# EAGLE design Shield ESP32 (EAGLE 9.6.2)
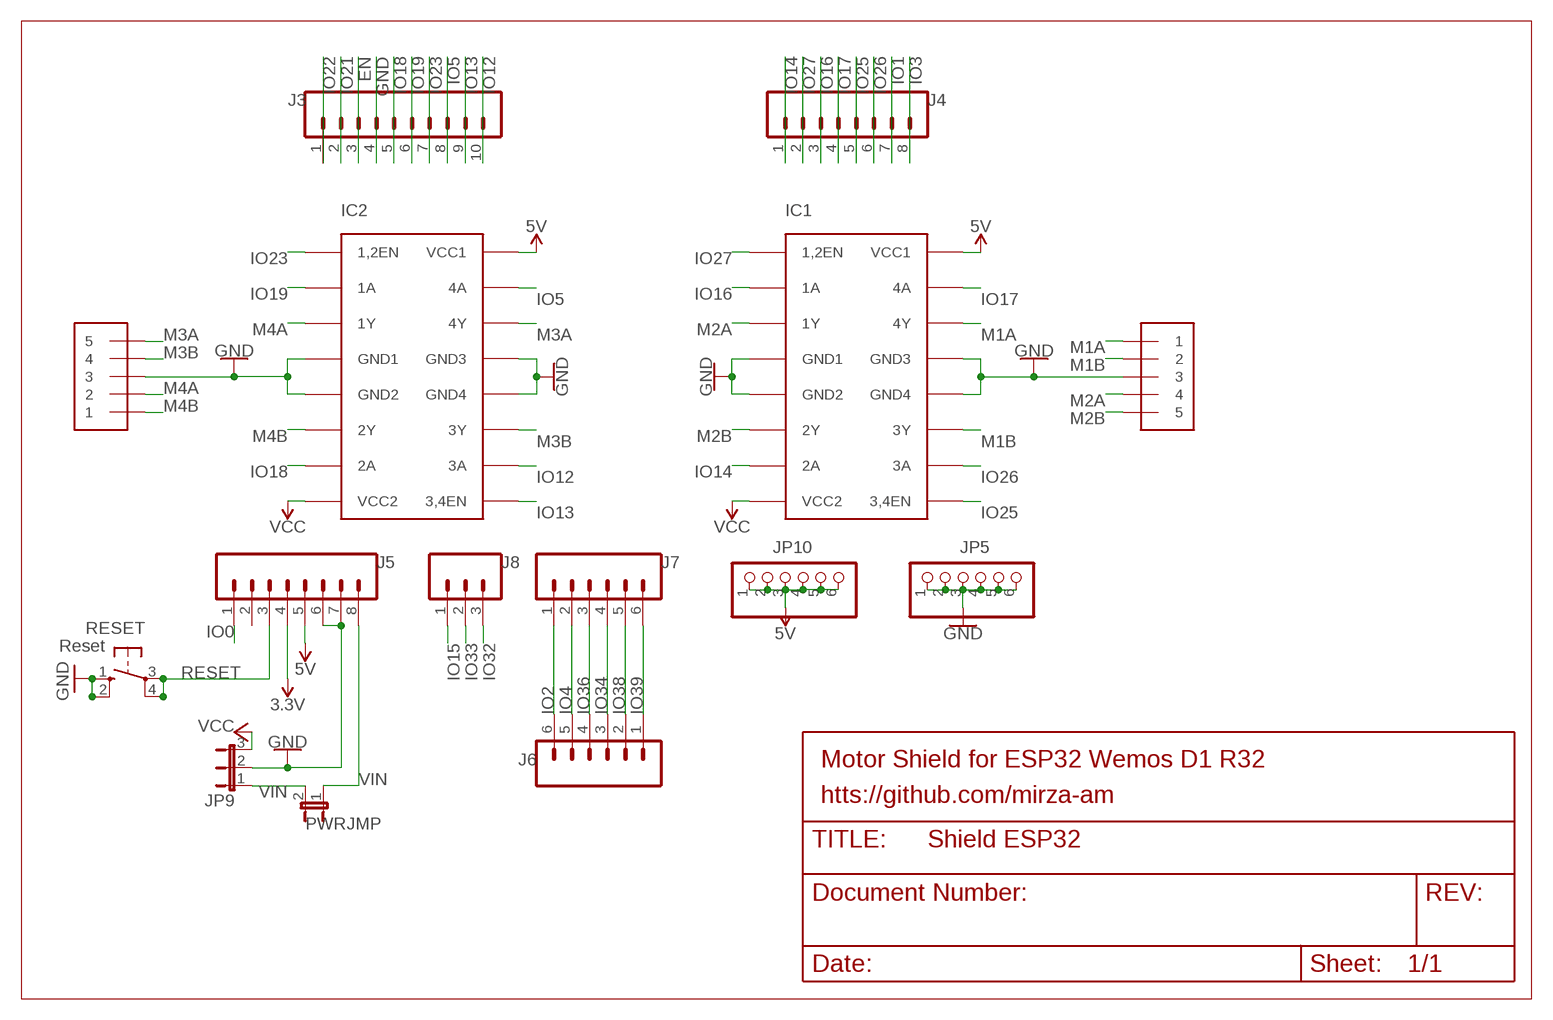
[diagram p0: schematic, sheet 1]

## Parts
IC1  L293D  [DIL16]
IC2  L293D  [DIL16]
J1  1X5  [1X05-3.5MM]
J2  1X5  [1X05-3.5MM]
J3  CONN_10NO_SILK_PTH_FEMALE  [1X10_NO_SILK]
J4  CONN_08NO_SILK_FEMALE_PTH  [1X08_NO_SILK]
J5  CONN_08NO_SILK_FEMALE_PTH  [1X08_NO_SILK]
J6  CONN_06NO_SILK_FEMALE_PTH  [1X06_NO_SILK]
J7  CONN_06NO_SILK_FEMALE_PTH  [1X06_NO_SILK]
J8  CONN_031X03_NO_SILK  [1X03_NO_SILK]
JP5  PINHD-1X6B  [1X06-BIG]
JP9  JP2E  [JP2]
JP10  PINHD-1X6B  [1X06-BIG]
PWRJMP  JP1E  [JP1]
RESET  Reset  10-XX  [B3F-10XX]

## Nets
3.3V: J5.4
5V: IC1.16(VCC1) IC2.16(VCC1) J5.5 JP10.1 JP10.2 JP10.3 JP10.4 JP10.5 JP10.6
EN: J3.3
GND: IC1.4(GND1) IC1.5(GND2) IC1.12(GND4) IC1.13(GND3) IC2.4(GND1) IC2.5(GND2) IC2.12(GND4) IC2.13(GND3) J1.3 J2.3 J3.4 J5.6 J5.7 JP5.1 JP5.2 JP5.3 JP5.4 JP5.5 JP5.6 JP9.2 RESET.1(S) RESET.2(S1)
IO0: J5.1
IO1: J4.7
IO2: J6.6 J7.1
IO3: J4.8
IO4: J6.5 J7.2
IO5: IC2.15(4A) J3.8
IO12: IC2.10(3A) J3.10
IO13: IC2.9(3,4EN) J3.9
IO14: IC1.7(2A) J4.1
IO15: J8.1
IO16: IC1.2(1A) J4.3
IO17: IC1.15(4A) J4.4
IO18: IC2.7(2A) J3.5
IO19: IC2.2(1A) J3.6
IO21: J3.2
IO22: J3.1
IO23: IC2.1(1,2EN) J3.7
IO25: IC1.9(3,4EN) J4.5
IO26: IC1.10(3A) J4.6
IO27: IC1.1(1,2EN) J4.2
IO32: J8.3
IO33: J8.2
IO34: J6.3 J7.4
IO36: J6.4 J7.3
IO38: J6.2 J7.5
IO39: J6.1 J7.6
M1A: IC1.14(4Y) J2.1
M1B: IC1.11(3Y) J2.2
M2A: IC1.3(1Y) J2.4
M2B: IC1.6(2Y) J2.5
M3A: IC2.14(4Y) J1.5
M3B: IC2.11(3Y) J1.4
M4A: IC2.3(1Y) J1.2
M4B: IC2.6(2Y) J1.1
RESET: J5.3 RESET.3(P) RESET.4(P1)
VCC: IC1.8(VCC2) IC2.8(VCC2) JP9.3
VIN: J5.8 JP9.1 PWRJMP.1 PWRJMP.2
Unconnected: J5.2

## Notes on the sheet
- Motor Shield for ESP32 Wemos D1 R32
- htts://github.com/mirza-am

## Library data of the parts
IC1 IC2 = L293D:L293D
J1 J2 = adafruit:1X5
J3 = SparkFun-Connectors:CONN_10: Multi connection point. Often used as Generic Header-pin footprint for 0.1 inch spaced/style header connections On any of the 0.1 inch spaced packages, you can populate with these: Break Away Headers - Straight (PRT-00116) Break Away Male Headers - Right Angle (PRT-00553) Female Headers (PRT-00115)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; PROD_ID: CONN-11563
J4 J5 = SparkFun-Connectors:CONN_08: Multi connection point. Often used as Generic Header-pin footprint for 0.1 inch spaced/style header connections On any of the 0.1 inch spaced packages, you can populate with these: Break Away Headers - Straight (PRT-00116) Break Away Male Headers - Right Angle (PRT-00553) Female Headers (PRT-00115)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; PROD_ID: CONN-08438
J6 J7 = SparkFun-Connectors:CONN_06: Multi connection point. Often used as Generic Header-pin footprint for 0.1 inch spaced/style header connections On any of the 0.1 inch spaced packages, you can populate with these: Break Away Headers - Straight (PRT-00116) Break Away Male Headers - Right Angle (PRT-00553) Female Headers (PRT-00115)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; PROD_ID: CONN-08437
J8 = SparkFun-Connectors:CONN_03: Multi connection point. Often used as Generic Header-pin footprint for 0.1 inch spaced/style header connections On any of the 0.1 inch spaced packages, you can populate with these: Break Away Headers - Straight (PRT-00116) Break Away Male Headers - Right Angle (PRT-00553) Female Headers (PRT-00115)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
JP5 JP10 = carduino:PINHD-1X6: PIN HEADER
JP9 = jumper:JP2E: JUMPER
PWRJMP = jumper:JP1E: JUMPER
RESET = switch-omron:10-XX: OMRON SWITCH

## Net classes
1 power: width 0.61 mm

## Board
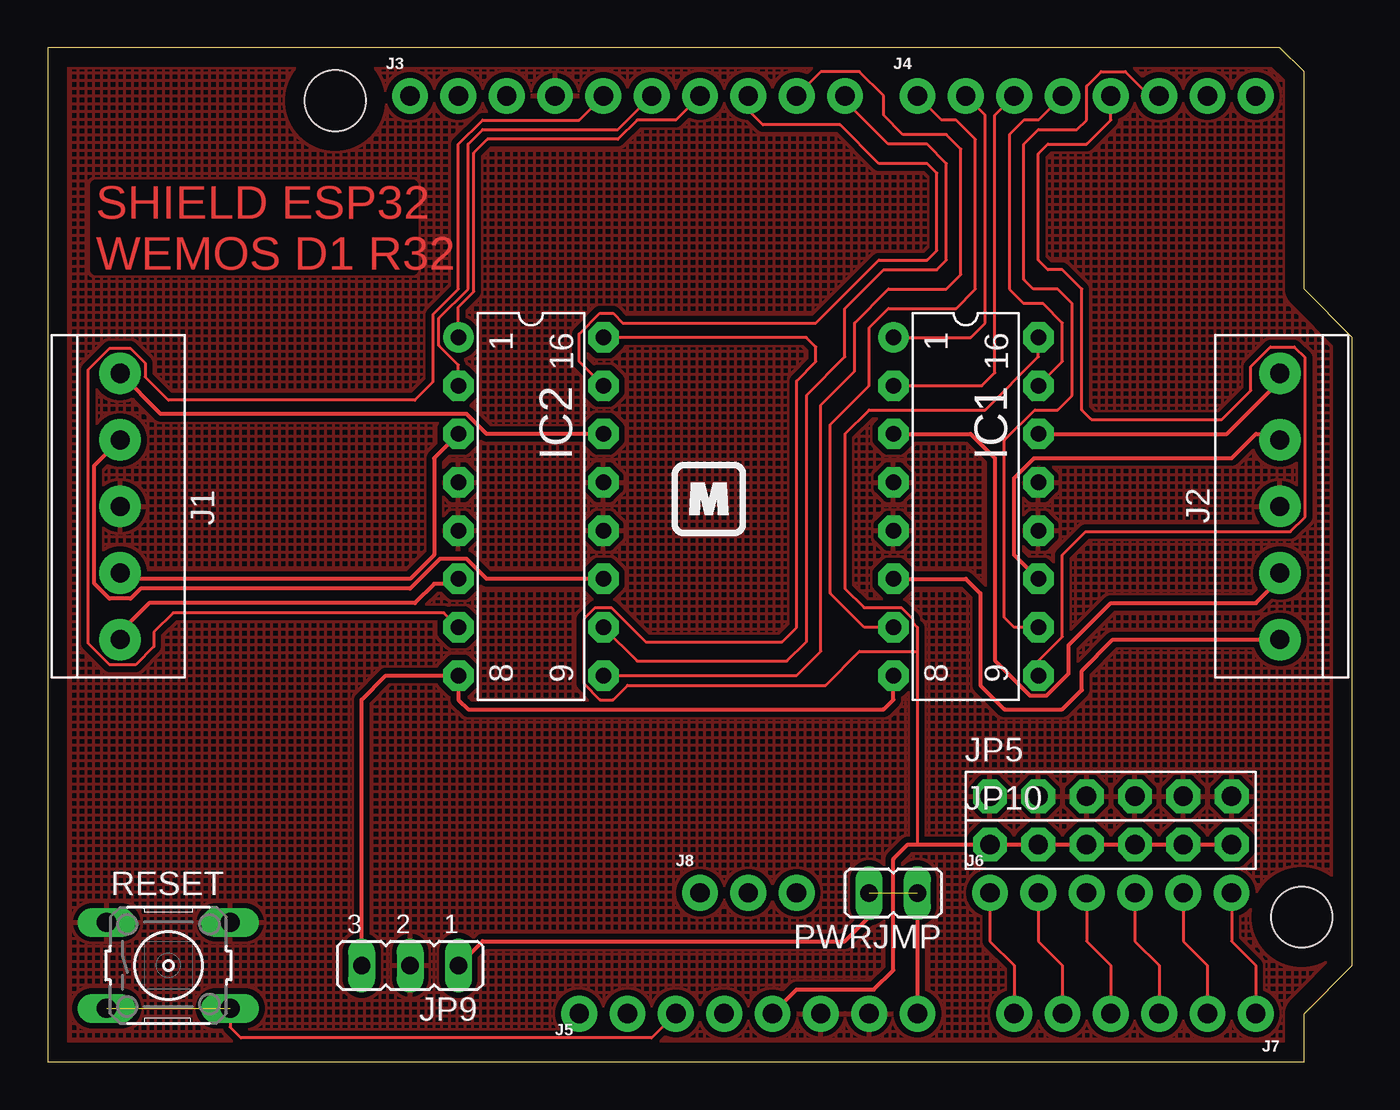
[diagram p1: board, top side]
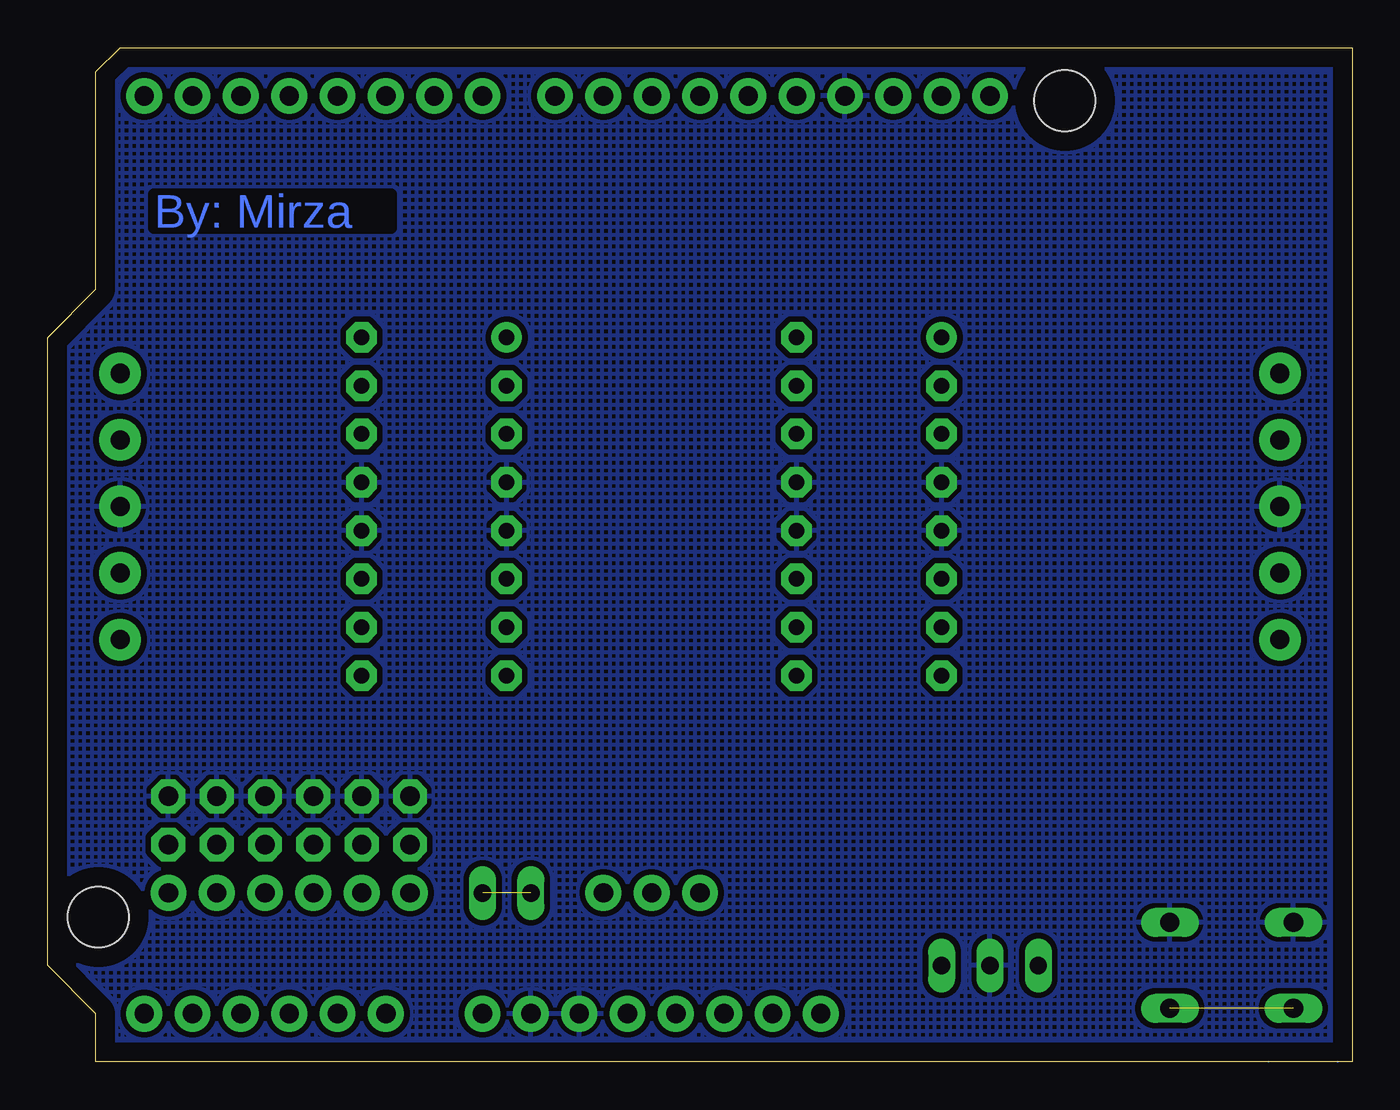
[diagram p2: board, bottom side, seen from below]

Size 68.58 x 53.34 mm. Coordinates in mm from the lower left corner, seen from the top.
Outline: 66.04,0 66.04,2.54 68.58,5.08 68.58,38.1 66.04,40.64 66.04,52.07 64.77,53.34 0,53.34 0,0 66.04,0
Copper layers (1*16): Top 0.035mm / dielectric 1.5mm / Bottom 0.035mm
Design rules "default": minimum track width 6mil, minimum drill 0.35mm, track to track 6mil, track to pad 6mil, pad to pad 6mil, via to via 6mil, smd to smd 6mil, copper to edge 40mil, drill to drill 6mil, minimum pad ring 10mil, minimum via ring 8mil, stop-mask expansion 4mil, vias tented up to drill 0mil, thermal gap 10mil
Holes 3.2 mm at 65.91,7.62 15.11,50.55

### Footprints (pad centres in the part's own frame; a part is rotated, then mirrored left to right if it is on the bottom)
DIL16 = drill 0.813 pad 1.6: 1 -8.89,-3.81 | drill 0.813 pad 1.6 octagon: 2 -6.35,-3.81; 3 -3.81,-3.81; 4 -1.27,-3.81; 5 1.27,-3.81; 6 3.81,-3.81; 7 6.35,-3.81; 8 8.89,-3.81; 9 8.89,3.81; 10 6.35,3.81; 11 3.81,3.81; 12 1.27,3.81; 13 -1.27,3.81; 14 -3.81,3.81; 15 -6.35,3.81; 16 -8.89,3.81
1X05-3.5MM = drill 1 pad 2.184: 1 7,0; 2 3.5,0; 3 0,0; 4 -3.5,0; 5 -7,0
1X10_NO_SILK = drill 1.016 pad 1.88: 1 0,0; 2 2.54,0; 3 5.08,0; 4 7.62,0; 5 10.16,0; 6 12.7,0; 7 15.24,0; 8 17.78,0; 9 20.32,0; 10 22.86,0
1X08_NO_SILK = drill 1.016 pad 1.88: 1 0,0; 2 2.54,0; 3 5.08,0; 4 7.62,0; 5 10.16,0; 6 12.7,0; 7 15.24,0; 8 17.78,0
1X06_NO_SILK = drill 1.016 pad 1.88: 1 0,0; 2 2.54,0; 3 5.08,0; 4 7.62,0; 5 10.16,0; 6 12.7,0
1X03_NO_SILK = drill 1.016 pad 1.88: 1 0,0; 2 2.54,0; 3 5.08,0
1X06-BIG = drill 1.016 pad 1.778 octagon: 1 -6.35,0; 2 -3.81,0; 3 -1.27,0; 4 1.27,0; 5 3.81,0; 6 6.35,0
JP2 = drill 0.914 long: 1 -2.54,0; 2 0,0; 3 2.54,0
JP1 = drill 0.914 long: 1 0,-1.27; 2 0,1.27
B3F-10XX = drill 1.016 long: 1 -3.251,2.261; 2 3.251,2.261; 3 -3.251,-2.261; 4 3.251,-2.261

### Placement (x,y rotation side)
IC1  48.26,29.21 270 top
IC2  25.4,29.21 270 top
J1  3.81,29.21 270 top
J2  64.77,29.21 90 top
J3  19.05,50.8 0 top
J4  45.72,50.8 0 top
J5  27.94,2.54 0 top
J6  49.53,8.89 0 top
J7  63.5,2.54 180 top
J8  34.29,8.89 0 top
JP5  55.88,13.97 0 top
JP9  19.05,5.08 180 top
JP10  55.88,11.43 0 top
PWRJMP  44.45,8.89 90 top
RESET  6.35,5.08 0 top
U$2  [LOGO_M2]  32.81,27.66 0 top

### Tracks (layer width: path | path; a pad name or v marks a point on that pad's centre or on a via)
5V
  Top 0.152: 45.72,21.59 45.72,22.86 45.48,23.1 45.48,23.29 44.88,23.89 42.91,23.89 41.91,24.89 41.91,33.02 43.18,34.29 49.28,34.29 52.07,37.08 IC1.16 | 45.72,21.59 42.67,21.59 40.89,19.81 30.48,19.81 29.72,19.05 29.02,19.05 28.18,19.89 28.18,23.29 28.78,23.89 29.64,23.89 31.43,22.1 38.61,22.1 39.37,22.86 39.37,35.81 40.39,36.83 40.39,37.59 39.88,38.1 IC2.16 | 45.72,21.59 45.72,11.43
  Top 0.203: J5.5 39.37,3.81 43.43,3.81 44.45,4.83 44.45,10.67 45.21,11.43 45.72,11.43 JP10.1 JP10.2 JP10.3 JP10.4 JP10.5 JP10.6
GND
  pour Top (isolate 0.305, hatched): 0,53.34 0,0 66.04,0 66.04,2.54 68.58,5.08 68.58,38.1 66.04,40.64 66.04,52.07 64.77,53.34
  pour Bottom (isolate 0.305, hatched): 0,53.34 0,0 66.04,0 66.04,2.54 68.58,5.08 68.58,38.1 66.04,40.64 66.04,52.07 64.77,53.34
IO2
  Top 0.152: J6.6 62.23,6.35 63.5,5.08 J7.1
IO4
  Top 0.152: J6.5 59.69,6.35 60.96,5.08 J7.2
IO5
  Top 0.152: IC2.15 27.94,36.83 27.94,38.28 29.02,39.37 29.72,39.37 30.23,38.86 40.39,38.86 43.69,42.16 46.23,42.16 46.74,42.67 46.74,46.74 46.23,47.24 43.69,47.24 41.66,49.28 37.59,49.28 36.83,50.04 J3.8
IO12
  Top 0.152: J3.10 41.91,50.55 44.2,48.26 46.23,48.26 47.24,47.24 47.24,42.16 46.74,41.66 43.94,41.66 41.91,39.62 41.91,37.08 39.88,35.05 39.88,22.1 38.86,21.08 30.99,21.08 IC2.10
IO13
  Top 0.152: J3.9 40.64,52.07 42.67,52.07 43.94,50.8 43.94,49.78 44.96,48.77 47.24,48.77 48.01,48.01 48.01,41.4 47.24,40.64 44.2,40.64 42.42,38.86 42.42,36.32 40.64,34.54 40.64,21.59 39.37,20.32 IC2.9
IO14
  Top 0.152: 44.2,22.86 IC1.7 42.93,22.86 41.15,24.64 41.15,33.53 43.18,35.56 43.18,38.61 44.2,39.62 47.75,39.62 48.77,40.64 48.77,48.51 47.75,49.53 46.99,49.53 J4.1
IO16
  Top 0.152: IC1.2 49.1,35.56 49.78,36.24 49.78,49.78 J4.3
IO17
  Top 0.152: IC1.15 53.34,36.83 53.34,38.86 52.32,39.88 51.31,39.88 50.55,40.64 50.55,48.77 51.31,49.53 52.07,49.53 J4.4
IO18
  Top 0.152: J3.5 27.94,49.53 22.86,49.53 21.59,48.26 21.59,40.64 20.26,39.31 20.26,35.75 19.3,34.8 6.35,34.8 5.13,36.02 5.13,36.76 4.36,37.53 3.26,37.53 2.13,36.4 2.13,22.02 3.26,20.89 4.63,20.89 5.59,21.84 5.59,22.61 6.6,23.62 20.83,23.62 IC2.7
IO19
  Top 0.152: IC2.2 21.59,36.65 20.56,37.67 20.56,39.1 22.1,40.64 22.1,48.26 22.86,49.02 29.97,49.02 J3.6
IO23
  Top 0.152: IC2.1 21.59,39.7 22.4,40.51 22.4,47.8 23.11,48.51 29.97,48.51 30.99,49.53 33.02,49.53 J3.7
IO25
  Top 0.152: IC1.9 52.07,21.08 53.34,22.35 53.34,26.67 54.56,27.89 65.32,27.89 66.09,28.66 66.09,37.03 65.53,37.59 64.26,37.59 63.25,36.58 63.25,35.31 61.72,33.78 54.86,33.78 54.36,34.29 54.36,40.64 53.34,41.66 52.58,41.66 52.07,42.16 52.07,47.75 52.58,48.26 54.61,48.26 55.88,49.53 J4.5
IO26
  Top 0.152: IC1.10 50.8,22.86 50.29,23.37 50.29,32.7 51.88,34.29 53.09,34.29 53.85,35.05 53.85,39.88 53.09,40.64 51.82,40.64 51.31,41.15 51.31,48.26 52.07,49.02 54.1,49.02 54.61,49.53 54.61,51.31 55.37,52.07 56.64,52.07 57.91,50.8 | 57.53,50.8 57.91,50.8 | 57.91,50.8 J4.6
IO27
  Top 0.152: IC1.1 48.51,38.1 49.28,38.86 49.28,49.78 J4.2
IO34
  Top 0.152: J6.3 54.61,6.35 55.88,5.08 J7.4
IO36
  Top 0.152: J6.4 57.15,6.35 58.42,5.08 J7.3
IO38
  Top 0.152: J6.2 52.07,6.35 53.34,5.08 J7.5
IO39
  Top 0.152: J6.1 49.53,6.35 50.8,5.08 J7.6
M1A
  Top 0.203: J2.1 64.77,36.07 64.77,35.81 61.98,33.02 IC1.14
M1B
  Top 0.203: IC1.11 50.8,26.67 50.8,30.7 51.85,31.75 62.23,31.75 63.5,33.02 64.46,33.02 J2.2
M2A
  Top 0.203: J2.4 64.77,25.4 63.5,24.13 55.88,24.13 53.67,21.92 53.67,20.43 52.51,19.27 51.63,19.27 51.2,19.7 51.02,19.88 49.78,21.11 49.78,31.75 48.51,33.02 IC1.3
M2B
  Top 0.203: IC1.6 48.26,25.4 49.02,24.64 49.02,19.81 50.29,18.54 53.34,18.54 54.36,19.56 54.36,20.57 55.99,22.21 J2.5
M3A
  Top 0.203: IC2.14 23.08,33.02 22.03,34.07 5.95,34.07 J1.5
M3B
  Top 0.203: IC2.11 23.08,25.4 22.03,26.45 20.61,26.45 19.05,24.89 4.9,24.89 4.37,24.36 3.25,24.36 2.46,25.15 2.46,31.36 J1.4
M4A
  Top 0.203: IC2.3 20.32,31.75 20.32,26.67 19.05,25.4 4.12,25.4 J1.2
M4B
  Top 0.203: IC2.6 21.34,25.15 20.32,25.15 19.3,24.13 5.33,24.13 3.81,22.61 J1.1
RESET  (1 unrouted)
  Top 0.152: RESET.4 9.6,1.83 10.16,1.27 31.75,1.27 J5.3
VCC
  Top 0.203: JP9.3 16.51,19.05 17.78,20.32 IC2.8 21.59,19.05 22.1,18.54 43.94,18.54 44.45,19.05 IC1.8
VIN  (1 unrouted)
  Top 0.203: PWRJMP.1 J5.8 | JP9.1 22.86,6.35 41.91,6.35 43.18,7.62 PWRJMP.2
(copper drawn outside any net)
  shapes: Bottom area x2, Top area x1

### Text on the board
Top: SHIELD ESP32 / WEMOS D1 R32
Bottom: By: Mirza
tStop: SHIELD ESP32 / WEMOS D1 R32
bStop: By: Mirza

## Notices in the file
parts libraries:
SparkFun-PowerSymbols: Licensing: Creative Commons ShareAlike 4.0 International - https://creativecommons.org/licenses/by-sa/4.0
